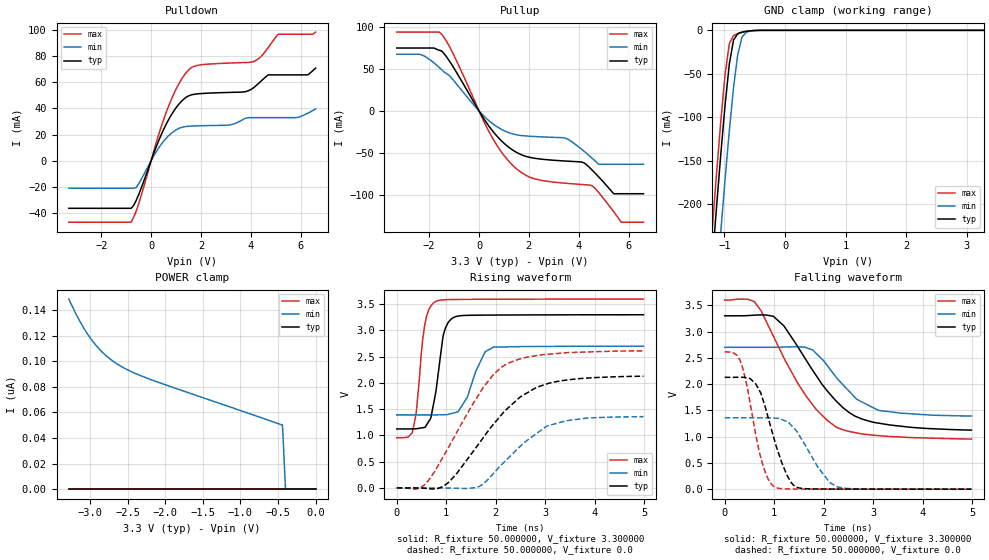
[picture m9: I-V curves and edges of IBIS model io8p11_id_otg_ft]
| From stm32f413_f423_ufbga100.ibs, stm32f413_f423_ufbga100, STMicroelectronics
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|   Model io8p11_id_otg_ft
[Model]  io8p11_id_otg_ft
Model_type I/O
Polarity   Non-Inverting
Enable   Active-Low
Vinl =   0.990000V
Vinh =   2.310000V
Vmeas =  1.650000V
Cref =   30.000000pF
Rref =   100.000000M
Vref =   0.0V
C_comp   2.283100pF   2.214400pF   2.357400pF
[Temperature Range]   25.000000   0.125000k   -40.000000
[Pullup Reference]   3.300000V   2.700000V   3.600000V
[Pulldown Reference]   0.0V   0.0V   0.0V
[POWER Clamp Reference]   3.300000V   2.700000V   3.600000V
[GND Clamp Reference]   0.0V   0.0V   0.0V
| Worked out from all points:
|   slope of the pulldown table from 0 to 0.495 V, typ, clamps not added: 20.9 ohm
|   slope of the pullup table from 0 to 0.495 V, typ, clamps not added: 22.6 ohm
|   GND clamp passes 1 mA (typ) near -0.62 V on its own axis
|   rising waveform, R_fixture 50.000000, V_fixture 3.300000: 20-80 % time 197ps typ, 331ps min, 162ps max; typ from 1.12 V to 3.3 V
|   rising waveform, R_fixture 50.000000, V_fixture 0.0: 20-80 % time 1.13ns typ, 947ps min, 998ps max; typ from 0 V to 2.13 V
|   falling waveform, R_fixture 50.000000, V_fixture 3.300000: 20-80 % time 1.01ns typ, 783ps min, 984ps max; typ from 3.3 V to 1.12 V
|   falling waveform, R_fixture 50.000000, V_fixture 0.0: 20-80 % time 415ps typ, 536ps min, 332ps max; typ from 2.13 V to 0 V
[Pulldown]
|Voltage   I(typ)   I(min)   I(max)
-3.3V     -36.46mA   -21.09mA   -47.09mA
-800mV    -36.46mA   -21.09mA   -47.09mA
-600mV    -30.5mA    -20.54mA   -38.68mA
700mV     31.4mA     19.11mA    41.71mA
1.2V      45.15mA    25.37mA    61.75mA
1.6V      50.35mA    26.5mA     71.06mA
3.1V      52.28mA    27.26mA    74.76mA
4.1V      55.71mA    33mA       75.81mA
4.7V      65.72mA    33mA       86.7mA
5.1V      65.72mA    33mA       96.91mA
6.3V      65.88mA    36.51mA    96.91mA
6.6V      70.94mA    39.72mA    98.51mA
[Pullup]
|Voltage   I(typ)   I(min)   I(max)
-3.3V     74.74mA    67.41mA    93.65mA
-2.3V     74.74mA    66.57mA    93.65mA
-1.5V     71.37mA    49mA       91.08mA
500mV     -22.07mA   -14mA      -30.03mA
1.6V      -50.64mA   -28.81mA   -70.96mA
3.5V      -59.53mA   -32.65mA   -85.92mA
4.2V      -61.43mA   -47.48mA   -87.46mA
4.5V      -69.06mA   -55.13mA   -88.38mA
4.8V      -78.22mA   -63.4mA    -96.84mA
5.4V      -98.3mA    -63.4mA    -119.6mA
5.7V      -98.3mA    -63.4mA    -132.1mA
6.6V      -98.3mA    -63.4mA    -132.1mA
[GND_clamp]
|Voltage   I(typ)   I(min)   I(max)
-3.3V     -2.316A    -2.396A    -2.289A
-1.2V     -265.5mA   -356.1mA   -227.2mA
-1.13V    -202.7mA   -292.9mA   -164.1mA
-1.06V    -142.2mA   -231.2mA   -104.1mA
-990mV    -85.98mA   -171.6mA   -50.73mA
-920mV    -38.81mA   -115.5mA   -15.3mA
-850mV    -11.1mA    -65.61mA   -6.021mA
-780mV    -3.796mA   -27.43mA   -3.892mA
-710mV    -2.096mA   -7.699mA   -2.393mA
-640mV    -1.154mA   -2.125mA   -1.227mA
-570mV    -528.1uA   -803.6uA   -480.7uA
3.28V     0A         0A         0A
[POWER_clamp]
|Voltage   I(typ)   I(min)   I(max)
-3.28V    0A         148.5nA    0A
-3.2V     0A         138.6nA    0A
-3.12V    0A         129.7nA    0A
-3.04V    0A         122nA      0A
-2.96V    0A         115.3nA    0A
-2.8V     0A         105.1nA    0A
-2.6V     0A         96.44nA    0A
-2.4V     0A         90.52nA    0A
-2.16V    0A         84.97nA    0A
-440mV    0A         50.04nA    0A
-400mV    0A         0A         0A
0V        0A         0A         0A
[Ramp]
| variable   typ   min   max
dV/dt_r  1.26150/1.11671n   0.80580/0.93825n   1.56072/0.99646n
dV/dt_f  1.27686/0.99427n   0.77058/0.75737n   1.57001/0.97645n
R_load = 50.000000
[Rising Waveform]
R_fixture= 50.000000
V_fixture= 3.300000
V_fixture_min= 2.700000
V_fixture_max= 3.600000
|time   V(typ)   V(min)   V(max)
0s        1.124V     1.392V     954.3mV
320.3ps   1.126V     1.392V     1.079V
390.4ps   1.128V     1.392V     1.413V
560.6ps   1.153V     1.392V     3.081V
690.7ps   1.344V     1.391V     3.469V
780.8ps   1.787V     1.391V     3.551V
951ps     2.951V     1.395V     3.585V
1.171ns   3.259V     1.435V     3.591V
1.952ns   3.294V     2.683V     3.595V
4.985ns   3.3V       2.7V       3.599V
[Rising Waveform]
R_fixture= 50.000000
V_fixture= 0.0
V_fixture_min= 0.0
V_fixture_max= 0.0
|time   V(typ)   V(min)   V(max)
0s        345.6uV    196.8uV    652.2uV
470.5ps   -2.82mV    136.3uV    -95.91uV
650.7ps   -14.06mV   197.3uV    155.2mV
951ps     37.15mV    -1.04mV    615.8mV
1.662ns   847.3mV    26.77mV    1.787V
2.182ns   1.468V     503.9mV    2.341V
2.503ns   1.738V     801.4mV    2.462V
3.033ns   1.983V     1.18V      2.546V
3.844ns   2.094V     1.332V     2.59V
4.985ns   2.129V     1.359V     2.612V
[Falling Waveform]
R_fixture= 50.000000
V_fixture= 3.300000
V_fixture_min= 2.700000
V_fixture_max= 3.600000
|time   V(typ)   V(min)   V(max)
0s        3.3V       2.7V       3.599V
600.6ps   3.312V     2.7V       3.567V
740.7ps   3.316V     2.7V       3.385V
981ps     3.292V     2.701V     2.917V
1.201ns   3.101V     2.705V     2.489V
1.772ns   2.271V     2.651V     1.613V
2.252ns   1.679V     2.13V      1.182V
2.673ns   1.374V     1.708V     1.069V
3.113ns   1.256V     1.499V     1.019V
4.985ns   1.124V     1.392V     954.3mV
[Falling Waveform]
R_fixture= 50.000000
V_fixture= 0.0
V_fixture_min= 0.0
V_fixture_max= 0.0
|time   V(typ)   V(min)   V(max)
0s        2.129V     1.359V     2.612V
310.3ps   2.129V     1.358V     2.454V
450.5ps   2.118V     1.358V     1.961V
630.6ps   1.998V     1.358V     1.022V
830.8ps   1.525V     1.36V      292.7mV
1.021ns   882.9mV    1.352V     35.81mV
1.401ns   68.01mV    1.159V     3.29mV
1.872ns   3.646mV    436.6mV    1.994mV
2.282ns   1.871mV    40.36mV    1.604mV
4.985ns   345.6uV    196.8uV    652.2uV
